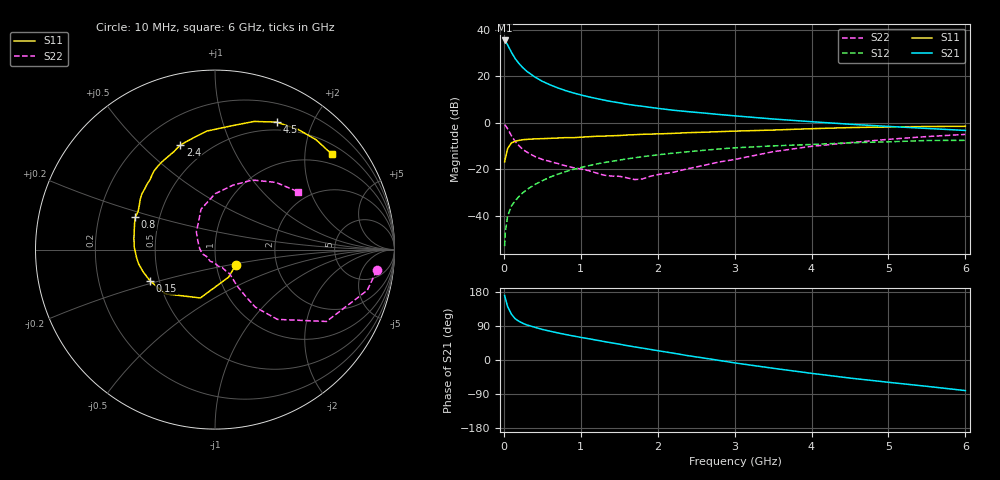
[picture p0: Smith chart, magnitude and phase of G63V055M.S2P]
! SIEMENS Small Signal Semiconductors
! BFG193
! Si NPN RF Bipolar Junction Transistor in SOT223
! VCE = 3 V  IC = 55 mA
! Common Emitter S-Parameters:  August  1996
# GHz  S  MA  R  50
!  f  S11  S21  S12  S22
! GHz  MAG  ANG  MAG  ANG  MAG  ANG  MAG  ANG
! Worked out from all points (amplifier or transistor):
!   36 points, 10 MHz to 6 GHz, reference 50 ohm
!   highest |S21| = 35.5 dB at 10 MHz (marker M1)
!   |S21| within 3 dB of that: start of sweep to 66.05 MHz
!   unconditionally stable (mu >= 1): 383.9 MHz to 2.375 GHz
!   at 250 MHz: K = 0.93, MSG = 26.8 dB, |S12| = -30.1 dB
!   at 1.4 GHz: K = 1.05, MAG = 11.6 dB, |S12| = -16.6 dB
!   at 6 GHz: K = 0.91, MSG = 2.1 dB, |S12| = -7.6 dB
!   S11 on the Smith chart (normalised r, x): 10 MHz: 1.24, -0.22; 150 MHz: 0.44, -0.18; 800 MHz: 0.36, +0.17; 2.4 GHz: 0.35, +0.66; 4.5 GHz: 0.40, +1.52; 6 GHz: 0.73, +2.64
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0.01  0.1442 -36.3  59.4 170.4  0.0022 82.2  0.909 -7.3
0.02  0.1711 -63.7  57.19 162.2  0.0046 79.9  0.8779 -15.0
0.05  0.2813 -106.8  47.33 140.5  0.0099 69.6  0.7391 -32.8
0.1  0.3711 -138.4  32.75 120.5  0.0164 68.3  0.5216 -48.2
0.15  0.4017 -154.4  23.79 108.4  0.0211 66.3  0.3912 -55.0
0.2  0.4189 -162.8  18.68 101.7  0.0262 69.0  0.3176 -56.6
0.25  0.4326 -169.3  15.2 96.5  0.0314 68.9  0.2641 -57.9
0.3  0.4391 -173.9  12.82 92.5  0.0364 69.7  0.2343 -58.6
0.4  0.4501 178.2  9.76 86.5  0.0465 69.8  0.1888 -58.7
0.5  0.456 172.1  7.839 80.7  0.0565 69.0  0.1625 -58.7
0.6  0.4624 166.6  6.586 76.1  0.0676 67.7  0.1467 -60.0
0.7  0.4704 162.4  5.662 71.6  0.078 66.2  0.133 -63.1
0.8  0.4797 157.9  4.95 67.4  0.0884 64.3  0.1187 -65.6
1.1  0.501 146.4  3.633 56.2  0.1189 58.9  0.0935 -79.5
1.3  0.5168 139.5  3.09 48.8  0.1388 54.8  0.0744 -92.0
1.6  0.5455 129.9  2.514 38.1  0.1673 47.9  0.0654 -121.5
2.2  0.5917 112.8  1.869 18.1  0.222 34.1  0.0859 175.7
2.4  0.6138 108.4  1.735 11.2  0.2384 29.8  0.1034 156.1
3.5  0.6973 82.0  1.208 -21.8  0.3182 2.5  0.2383 109.0
4.5  0.7888 64.2  0.931 -47.7  0.3714 -17.6  0.3735 74.3
5.5  0.8316 47.4  0.757 -69.5  0.4152 -40.9  0.5054 47.8
6  0.8406 39.1  0.684 -80.7  0.4191 -54.3  0.5625 35.1
